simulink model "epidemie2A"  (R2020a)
settings: Solver=FixedStepDiscrete  StartTime=0.0  StopTime=300  FixedStep=1  RelTol=1e-3  EnableMultiTasking=on
InitFcn:
  | init_epidemie
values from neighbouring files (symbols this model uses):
  alpha = 2e-6    (= 2e-06)    [init_epidemie.m]
  beta = 1    [init_epidemie.m]
  delta = 0.1    [init_epidemie.m]
  epsilon = 5e-3    (= 0.005)    [init_epidemie.m]
  gamma = 0.9    [init_epidemie.m]
  zeta = 4e-3    (= 0.004)    [init_epidemie.m]

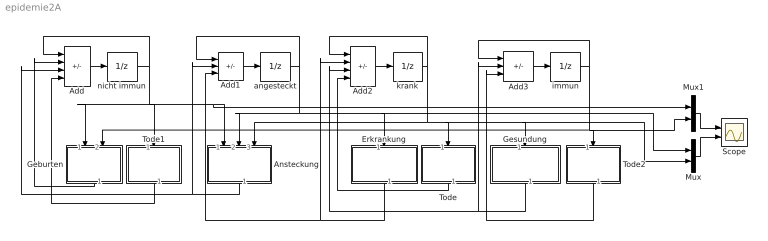
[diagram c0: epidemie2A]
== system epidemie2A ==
  Add : Sum  Inputs=++--
  Add1 : Sum  Inputs=++-
  Add2 : Sum  Inputs=++--
  Add3 : Sum  Inputs=++-
  Ansteckung : Subsystem
  Erkrankung : Subsystem
  Geburten : Subsystem
  Gesundung : Subsystem
  Mux : Mux  Inputs=2
  Mux1 : Mux  Inputs=2
  Scope : Scope  NumInputPorts=2
  Tode : Subsystem
  Tode1 : Subsystem
  Tode2 : Subsystem
  angesteckt : UnitDelay  InitialCondition=1  SampleTime=-1  HasFrameUpgradeWarning=on
  immun : UnitDelay  SampleTime=-1  HasFrameUpgradeWarning=on
  krank : UnitDelay  SampleTime=-1  HasFrameUpgradeWarning=on
  nicht immun : UnitDelay  InitialCondition=1e6  SampleTime=-1  HasFrameUpgradeWarning=on
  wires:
  Add/1 -> nicht immun/1
  nicht immun/1 -> Add/1, Ansteckung/1(N), Mux1/1, Tode1/1(N), Geburten/1(N)
  immun/1 -> Add3/1, Mux1/2, Tode2/1(I), Geburten/2(I)
  Geburten/1(b) -> Add/2
  angesteckt/1 -> Add1/1, Ansteckung/2(A), Erkrankung/1(A), Mux/1
  krank/1 -> Ansteckung/3(K), Tode/1(K), Gesundung/1(K), Mux/2, Add2/1
  Ansteckung/1(a) -> Add/3, Add1/2
  Add1/1 -> angesteckt/1
  Erkrankung/1(k) -> Add1/3, Add2/2
  Add2/1 -> krank/1
  Gesundung/1(g) -> Add2/3, Add3/2
  Tode/1(t) -> Add2/4
  Mux1/1 -> Scope/1
  Mux/1 -> Scope/2
  Add3/1 -> immun/1
  Tode2/1(di) -> Add3/3
  Tode1/1(dn) -> Add/4

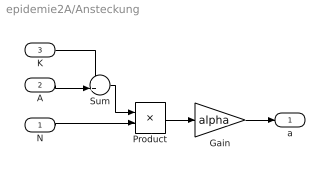
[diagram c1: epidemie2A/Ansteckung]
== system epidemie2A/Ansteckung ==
  N : Inport
  A : Inport  Port=2
  K : Inport  Port=3
  Gain : Gain  Gain=alpha
  Product : Product  RndMeth=Zero
  Sum : Sum  Inputs=++|
  a : Outport
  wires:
  Sum/1 -> Product/1
  Product/1 -> Gain/1
  K/1 -> Sum/1
  A/1 -> Sum/2
  Gain/1 -> a/1
  N/1 -> Product/2

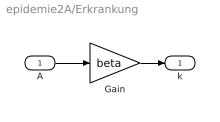
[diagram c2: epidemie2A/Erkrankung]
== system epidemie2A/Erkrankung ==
  A : Inport
  Gain : Gain  Gain=beta
  k : Outport
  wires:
  A/1 -> Gain/1
  Gain/1 -> k/1

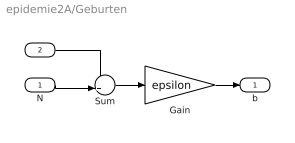
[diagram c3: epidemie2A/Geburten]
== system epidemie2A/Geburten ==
  N : Inport
  I : Inport  Port=2
  Gain : Gain  Gain=epsilon
  Sum : Sum  Inputs=++|
  b : Outport
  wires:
  Gain/1 -> b/1
  Sum/1 -> Gain/1
  N/1 -> Sum/2
  I/1 -> Sum/1

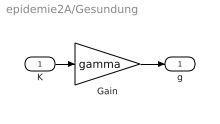
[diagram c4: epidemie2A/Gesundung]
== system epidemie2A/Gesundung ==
  K : Inport
  Gain : Gain  Gain=gamma
  g : Outport
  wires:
  Gain/1 -> g/1
  K/1 -> Gain/1

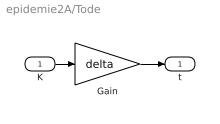
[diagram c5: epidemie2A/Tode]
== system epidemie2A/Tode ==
  K : Inport
  Gain : Gain  Gain=delta
  t : Outport
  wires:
  K/1 -> Gain/1
  Gain/1 -> t/1

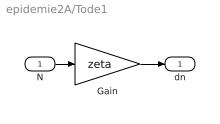
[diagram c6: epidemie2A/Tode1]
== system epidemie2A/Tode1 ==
  N : Inport
  Gain : Gain  Gain=zeta
  dn : Outport
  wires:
  Gain/1 -> dn/1
  N/1 -> Gain/1

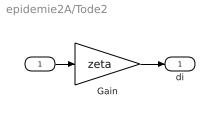
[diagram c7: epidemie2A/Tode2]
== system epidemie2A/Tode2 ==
  I : Inport
  Gain : Gain  Gain=zeta
  di : Outport
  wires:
  I/1 -> Gain/1
  Gain/1 -> di/1
